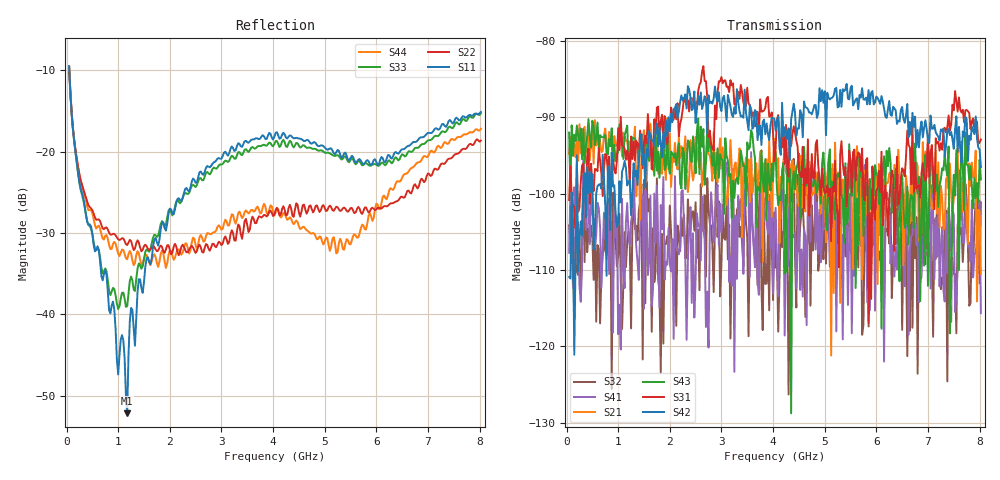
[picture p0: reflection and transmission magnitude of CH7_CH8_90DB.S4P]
!Agilent Technologies,E5071C,MY46316741,A.11.02
!Date: Mon Jun 01 10:26:07 2026
!Data & Calibration Information:
!1:CH7 INPUT 2:CH7 OUTPUT 3:CH8 INPUT 4:CH8 OUTPUT
!Freq	S11:SOLT4(ON)	S12:SOLT4(ON)	S13:SOLT4(ON)	S14:SOLT4(ON)
!	S21:SOLT4(ON)	S22:SOLT4(ON)	S23:SOLT4(ON)	S24:SOLT4(ON)
!	S31:SOLT4(ON)	S32:SOLT4(ON)	S33:SOLT4(ON)	S34:SOLT4(ON)
!	S41:SOLT4(ON)	S42:SOLT4(ON)	S43:SOLT4(ON)	S44:SOLT4(ON)
!PortZ  Port1:50+j0  Port2:50+j0  Port3:50+j0  Port4:50+j0
!Above PortZ is port z conversion or system Z0 setting when saving the data.
!When reading, reference impedance value at option line is always used.
# Hz S dB R 50
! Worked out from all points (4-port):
!   320 points, 50 MHz to 8.025 GHz, reference 50 ohm
!   strongest paths, dB at 50 MHz, 2.05 GHz, 4.05 GHz, 6.05 GHz, 8.025 GHz:
!     S42: -110.9, -90.7, -91.8, -87.8, -96.5
!     S31: -100.8, -89.6, -93.9, -97.0, -92.9
!     S43: -92.0, -94.7, -94.8, -101.4, -98.2
!     S21: -94.8, -95.3, -94.4, -96.1, -110.5
!     S41: -107.8, -105.9, -101.9, -102.3, -115.7
!     S32: -104.2, -109.3, -109.7, -108.7, -101.1
!   lowest |S11| = -52.2 dB at 1.175 GHz (marker M1), VSWR 1.00, Z = 49.8 - j0.174 ohm
!   |S11| at or under -10 dB: 53.76 MHz to end of sweep
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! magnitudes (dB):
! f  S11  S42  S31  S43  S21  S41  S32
! 50 MHz  -9.5  -110.9  -100.8  -92.0  -94.8  -107.8  -104.2
! 400 MHz  -28.7  -96.6  -95.1  -92.5  -94.7  -98.7  -107.7
! 1.175 GHz  -52.2  -98.9  -94.3  -91.1  -93.1  -101.3  -106.4
! 1.4 GHz  -35.7  -95.7  -94.2  -96.0  -94.6  -111.3  -102.2
! 2.575 GHz  -22.5  -88.4  -85.8  -97.5  -96.6  -104.4  -112.6
! 5.225 GHz  -20.1  -86.2  -101.2  -98.3  -99.7  -118.0  -111.9
! 8.025 GHz  -15.1  -96.5  -92.9  -98.2  -110.5  -115.7  -101.1
